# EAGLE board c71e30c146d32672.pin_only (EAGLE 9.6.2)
REV: C

Size 59.69 x 104.14 mm. Coordinates in mm from the lower left corner, seen from the top.
Outline: 0,101.6 0,2.54 arc90 2.54,0 57.15,0 arc90 59.69,2.54 59.69,101.6 arc90 57.15,104.14 2.54,104.14 arc90 0,101.6
Copper layers (1*16): Top 0.035mm / dielectric 1.5mm / Bottom 0.035mm
Design rules "adafruit 7-7": minimum track width 7mil, minimum drill 15.5mil, track to track 7mil, track to pad 7mil, pad to pad 7mil, via to via 7mil, smd to smd 7mil, copper to edge 10mil, drill to drill 8mil, minimum pad ring 10mil, minimum via ring 8mil, stop-mask expansion 2mil, vias tented up to drill 20mil, thermal gap 10mil
Net classes: 0 default: width 0.178 mm; 1 power: width 0.254 mm; 2 5V: width 0.406 mm, drill 0.483 mm
tRestrict: area 35.6,75.7 to 47.8,80
bRestrict: area 35.6,75.7 to 47.8,80

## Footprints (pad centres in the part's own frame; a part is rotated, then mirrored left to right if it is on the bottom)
0603-NO = smd 1.075 x 1: 1 -0.85,0; 2 0.85,0
0805-NO = smd 1.24 x 1.5: 1 -0.95,0; 2 0.95,0
JST_SH4 = smd 0.6 x 1.55: 1 -1.5,2.514; 2 -0.5,2.514; 3 0.5,2.514; 4 1.5,2.514 | smd 1.2 x 1.8: MT1 -2.8,-1.386; MT2 2.8,-1.386
SOD-323 = smd 1.35 x 0.8: A 1.27,0; C -1.27,0
SOT23-5 = smd 0.69 x 0.99: 1 -0.95,-1.29; 2 0,-1.29; 3 0.95,-1.29; 4 0.95,1.3; 5 -0.95,1.3
SOT23-6 = smd 0.55 x 1.2: 1 -0.95,-1.3; 2 0,-1.3; 3 0.95,-1.3; 4 0.95,1.3; 5 0,1.3; 6 -0.95,1.3
QFN56_7MM_REDUCEDEPAD = smd 0.875 x 0.2: 1 -3.45,2.6; 2 -3.45,2.2; 3 -3.45,1.8; 4 -3.45,1.4; 5 -3.45,1; 6 -3.45,0.6; 7 -3.45,0.2; 8 -3.45,-0.2; 9 -3.45,-0.6; 10 -3.45,-1; 11 -3.45,-1.4; 12 -3.45,-1.8; 13 -3.45,-2.2; 14 -3.45,-2.6; 29 3.45,-2.6; 30 3.45,-2.2; 31 3.45,-1.8; 32 3.45,-1.4; 33 3.45,-1; 34 3.45,-0.6; 35 3.45,-0.2; 36 3.45,0.2; 37 3.45,0.6; 38 3.45,1; 39 3.45,1.4; 40 3.45,1.8; 41 3.45,2.2; 42 3.45,2.6 | smd 0.2 x 0.875: 15 -2.6,-3.45; 16 -2.2,-3.45; 17 -1.8,-3.45; 18 -1.4,-3.45; 19 -1,-3.45; 20 -0.6,-3.45; 21 -0.2,-3.45; 22 0.2,-3.45; 23 0.6,-3.45; 24 1,-3.45; 25 1.4,-3.45; 26 1.8,-3.45; 27 2.2,-3.45; 28 2.6,-3.45; 43 2.6,3.45; 44 2.2,3.45; 45 1.8,3.45; 46 1.4,3.45; 47 1,3.45; 48 0.6,3.45; 49 0.2,3.45; 50 -0.2,3.45; 51 -0.6,3.45; 52 -1,3.45; 53 -1.4,3.45; 54 -1.8,3.45; 55 -2.2,3.45; 56 -2.6,3.45 | smd 3.2 x 3.2: P$1 0,0
CHIPLED_0603_NOOUTLINE = smd 0.8 x 0.8: A 0,-0.75; C 0,0.75
NEO3535_REVERSE = smd 1.2 x 0.9 bottom: 1-VDD 2.65,-0.75; 2-DOUT 2.65,0.75; 3-GND -2.65,0.75; 4-DIN -2.65,-0.75
RESPACK_4X0603 = smd 0.45 x 0.9: 1 -1.3,-0.85; 2 -0.4,-0.85; 3 0.4,-0.85; 4 1.3,-0.85; 5 1.3,0.85; 6 0.4,0.85; 7 -0.4,0.85; 8 -1.3,0.85
BUZZER_SMT_7.5MM = smd 2 x 2: + 2.8,-2.8; - 2.8,2.8; MT2 -2.8,2.8 | smd 2 x 1 rotated 135: MT -3,-3
PEC11+SWITCH = drill 1 pad 1.8: P$1 -2.54,7.62; P$2 2.54,7.62; P$A -2.54,-7.62; P$B 2.54,-7.62; P$C 0,-7.62 | drill 1.8 pad 2.8 long: P$GND1 -6.35,0; P$GND2 6.35,0
SPST_TACTILE_RA = smd 1.1 x 1.5: 1 -2.1,0.9; 2 2.1,0.9 | smd 1.75 x 1: MT1 -3.175,-0.9; MT2 3.075,-0.9 | hole 1: -1.15,-0.3; 1.15,-0.3
SMT_NUT_3MM = drill 4.25 pad 4.572: P$1 0,0
TESTPOINT_ROUND_1.5MM_NO = smd 1.5 x 1.5: P$1 0,0
USON8_4X4 = smd 0.6 x 0.4: 1 -1.85,1.2; 2 -1.85,0.4; 3 -1.85,-0.4; 4 -1.85,-1.2; 5 1.85,-1.2; 6 1.85,-0.4; 7 1.85,0.4; 8 1.85,1.2 | smd 2 x 3: PAD 0,0
SOT23-5' = smd 0.55 x 1.2: 1 -0.95,-1.3; 2 0,-1.3; 3 0.95,-1.3; 4 0.95,1.3; 5 -0.95,1.3
KAILH_SOCKET = smd 2.55 x 2.5 bottom: 1 6.09,5.08; 2 -7.36,2.5 | hole 3.9: 0,0 | hole 3.2: 2.54,5.08; -3.81,2.54 | hole 1.813: 5.08,0; -5.08,0
FIDUCIAL_1MM = smd 1 x 1: 1 0,0
USB_C_CUSB31-CFM2AX-01-X = smd 0.575 x 1.15: A1B12 -3.2,3.545; A4B9 -2.4,3.545; B1A12 3.2,3.545; B4A9 2.4,3.545 | smd 0.275 x 1.15: A5 -1.25,3.545; A6 -0.25,3.545; A7 0.25,3.545; A8 1.25,3.545; B5 1.75,3.545; B6 0.75,3.545; B7 -0.75,3.545; B8 -1.75,3.545 | drill 0.6 pad 1 long: M1 -4.32,2.97; M2 4.32,2.97; M3 -4.32,-1.21; M4 4.32,-1.21 | hole 0.65: 2.89,2.47; -2.89,2.47
ZJY130-2864KSWLG22 = smd 0.3 x 1.4 bottom: 1 -3.75,6.728; 2 -3.25,6.728; 3 -2.75,6.728; 4 -2.25,6.728; 5 -1.75,6.728; 6 -1.25,6.728; 7 -0.75,6.728; 8 -0.25,6.728; 9 0.25,6.728; 10 0.75,6.728; 11 1.25,6.728; 12 1.75,6.728; 13 2.25,6.728; 14 2.75,6.728; 15 3.25,6.728; 16 3.75,6.728 | smd 1.8 x 2.2 bottom: SUPPORT1 5.7,4.1; SUPPORT2 -5.7,4.1
CRYSTAL_2.5X2 = smd 0.9 x 0.75: 1 -0.825,-0.625; 2 0.825,-0.625; 3 0.825,0.625; 4 -0.825,0.625

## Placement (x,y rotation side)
C1  1uF  [0603-NO]  37.72,88.52 0 top
C2  1uF  [0603-NO]  35.18,91.19 90 top
C3  0.1uF  [0603-NO]  33.02,78.17 90 top
C4  0.1uF  [0603-NO]  30.86,92.71 270 top
C5  0.1uF  [0603-NO]  25.4,89.28 180 top
C6  10µF  [0805-NO]  46.73,85.56 90 top
C7  10uF  [0805-NO]  49.4,89.92 90 top
C8  10µF  [0805-NO]  40.59,84.14 270 top
C9  10uF  [0805-NO]  40.51,102.36 180 top
C10  0.1uF  [0603-NO]  24.38,83.57 180 top
C11  1uF  [0603-NO]  33.66,92.58 90 top
C12  0.1uF  [0603-NO]  38.86,84.2 270 top
C13  0.1uF  [0603-NO]  36.7,90.81 90 top
C14  10uF  [0805-NO]  36.7,102.36 0 top
C15  1uF  [0603-NO]  45.85,89.79 90 top
C16  0.1uF  [0603-NO]  23.37,97.03 180 top
C17  1uF  [0603-NO]  47.62,89.79 90 top
C18  0.1uF  [0603-NO]  37.66,67.94 270 top
C19  12pF  [0603-NO]  25.65,75.31 0 top
C20  12pF  [0603-NO]  29.84,77.22 90 top
C21  0.1uF  [0603-NO]  43.69,89.92 90 top
C22  10uF  [0805-NO]  23.37,33.91 0 top
C23  10uF  [0805-NO]  23.37,15.11 0 top
C24  10uF  [0805-NO]  43.56,72.07 0 top
C25  10uF  [0805-NO]  23.24,53.09 0 top
C26  0.1uF  [0603-NO]  23.37,32.26 180 top
C27  0.1uF  [0603-NO]  23.37,13.34 180 top
C28  0.1uF  [0603-NO]  23.24,51.44 180 top
C29  0.1uF  [0603-NO]  43.5,70.55 180 top
C30  10nF  [0603-NO]  40.13,70.55 180 top
C31  0.1uF  [0603-NO]  31.37,77.22 90 top
CONN1  STEMMA_I2C_QT  [JST_SH4]  57.15,92.71 90 top
D3  1N4148  [SOD-323]  22.86,89.53 90 top
IC1  74HCT1G125DBV  [SOT23-5]  54.48,73.15 180 top
IC2  PAM8301  [SOT23-6]  39.75,62.23 90 top
IC3  RP2040_QFN56  [QFN56_7MM_REDUCEDEPAD]  31.24,85.85 0 top
L  RED  [CHIPLED_0603_NOOUTLINE]  22.99,103.25 90 top
LED1  WS2812B_SK6812E  [NEO3535_REVERSE]  48.9,72.9 0 bottom
LED2  WS2812B_SK6812E  [NEO3535_REVERSE]  29.84,72.9 0 bottom
LED3  WS2812B_SK6812E  [NEO3535_REVERSE]  10.79,72.9 0 bottom
LED4  WS2812B_SK6812E  [NEO3535_REVERSE]  48.9,53.98 0 bottom
LED5  WS2812B_SK6812E  [NEO3535_REVERSE]  29.84,53.85 0 bottom
LED6  WS2812B_SK6812E  [NEO3535_REVERSE]  10.79,53.85 0 bottom
LED7  WS2812B_SK6812E  [NEO3535_REVERSE]  48.9,34.8 0 bottom
LED8  WS2812B_SK6812E  [NEO3535_REVERSE]  29.84,34.67 0 bottom
LED9  WS2812B_SK6812E  [NEO3535_REVERSE]  10.79,34.8 0 bottom
LED10  WS2812B_SK6812E  [NEO3535_REVERSE]  48.9,15.75 0 bottom
LED11  WS2812B_SK6812E  [NEO3535_REVERSE]  29.84,15.88 0 bottom
LED12  WS2812B_SK6812E  [NEO3535_REVERSE]  10.79,15.62 0 bottom
R1  5.1K  [RESPACK_4X0603]  23.11,100.2 270 top
R2  10k  [0603-NO]  23.37,95.5 180 top
R3  22  [0603-NO]  29.72,95.5 0 top
R4  22  [0603-NO]  32.77,95.5 180 top
R5  47K  [0603-NO]  39.24,65.53 270 top
R6  1K  [0603-NO]  29.21,79.5 0 top
R7  10K  [0603-NO]  57.15,74.36 90 top
R8  1K  [0603-NO]  37.66,71.37 270 top
R9  DNP  [0603-NO]  40.13,68.9 180 top
R10  10K  [0603-NO]  24.7,77.72 270 top
R11  1K  [0603-NO]  22.78,93.18 270 top
R12  680K  [0603-NO]  38.61,90.81 90 top
R14  5.1K  [RESPACK_4X0603]  50.04,94.61 90 top
SP2  7.5mm SPK  [BUZZER_SMT_7.5MM]  39.37,56.52 90 top
SW1  PEC11  [PEC11+SWITCH]  11.43,90.17 45 bottom
SW2  RA SW  [SPST_TACTILE_RA]  57.91,84.45 90 top
TP1  SEWTAP_SMTNUTM3  [SMT_NUT_3MM]  3.81,19.05 0 top
TP2  SEWTAP_SMTNUTM3  [SMT_NUT_3MM]  55.88,19.05 0 top
TP3  SEWTAP_SMTNUTM3  [SMT_NUT_3MM]  3.81,100.33 0 top
TP4  SEWTAP_SMTNUTM3  [SMT_NUT_3MM]  55.88,100.33 0 top
TP5  [TESTPOINT_ROUND_1.5MM_NO]  49.53,80.01 0 top
TP6  [TESTPOINT_ROUND_1.5MM_NO]  20.83,95.5 0 top
U1  GD25x16  [USON8_4X4]  26.91,92.71 0 top
U2  AP2112K-3.3  [SOT23-5']  43.56,85.72 90 top
U$1  SOCKET  [KAILH_SOCKET]  48.9,10.79 180 bottom
U$2  SOCKET  [KAILH_SOCKET]  29.84,10.79 180 bottom
U$3  SOCKET  [KAILH_SOCKET]  10.79,10.79 180 bottom
U$4  SOCKET  [KAILH_SOCKET]  10.79,29.84 180 bottom
U$5  SOCKET  [KAILH_SOCKET]  29.84,29.84 180 bottom
U$6  SOCKET  [KAILH_SOCKET]  48.9,29.84 180 bottom
U$12  SOCKET  [KAILH_SOCKET]  10.79,67.94 180 bottom
U$13  SOCKET  [KAILH_SOCKET]  29.84,67.94 180 bottom
U$34  FIDUCIAL_1MM  [FIDUCIAL_1MM]  50.93,102.23 0 top
U$35  FIDUCIAL_1MM  [FIDUCIAL_1MM]  3.31,3.1 0 top
U$40  SOCKET  [KAILH_SOCKET]  48.9,67.94 180 bottom
U$41  SOCKET  [KAILH_SOCKET]  10.79,48.9 180 bottom
U$42  SOCKET  [KAILH_SOCKET]  29.84,48.9 180 bottom
U$43  SOCKET  [KAILH_SOCKET]  48.9,48.9 180 bottom
U$78  [MACROPAD_TOP]  59.44,0.51 0 bottom
U$79  [MACROPAD_BOTTOM]  0,0 0 top
U$80  FIDUCIAL_1MM  [FIDUCIAL_1MM]  56.64,13.72 0 top
U$81  [PCBFEAT-REV-040]  50.04,97.92 0 top
X1  TYPE C  [USB_C_CUSB31-CFM2AX-01-X]  29.84,101.47 180 top
X2  ZJY130-2864KSWLG22  [ZJY130-2864KSWLG22]  41.66,93.41 0 bottom
Y1  12MHZ  [CRYSTAL_2.5X2]  27.56,77.34 180 top

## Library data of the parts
C1-C7 C9-C31 CONN1 D3 IC2 L LED1-LED12 R1-R12 R14 SP2 TP5 TP6 U1 U2 Y1 = microbuilder
C8 = microbuilder; COMPANY: ADAFRUIT INDUSTRIES; DRAWN: KTOWN; REV: C
IC1 = 74xx-little-us
IC3 = adafruit_micro
SW1 SW2 TP1-TP4 U$1-U$6 U$12 U$13 U$40-U$43 X1 = adafruit_electromech
U$34 U$35 U$80 = microbuilder; BOM: EXCLUDE
U$78 U$79 = keeb_silks
U$81 = microbuilder; REV: C
X2 = adafruit_display

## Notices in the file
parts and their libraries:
microbuilder: This work is placed in the public domain, and may be freely used for commercial and non-commercial work with the following conditions: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
